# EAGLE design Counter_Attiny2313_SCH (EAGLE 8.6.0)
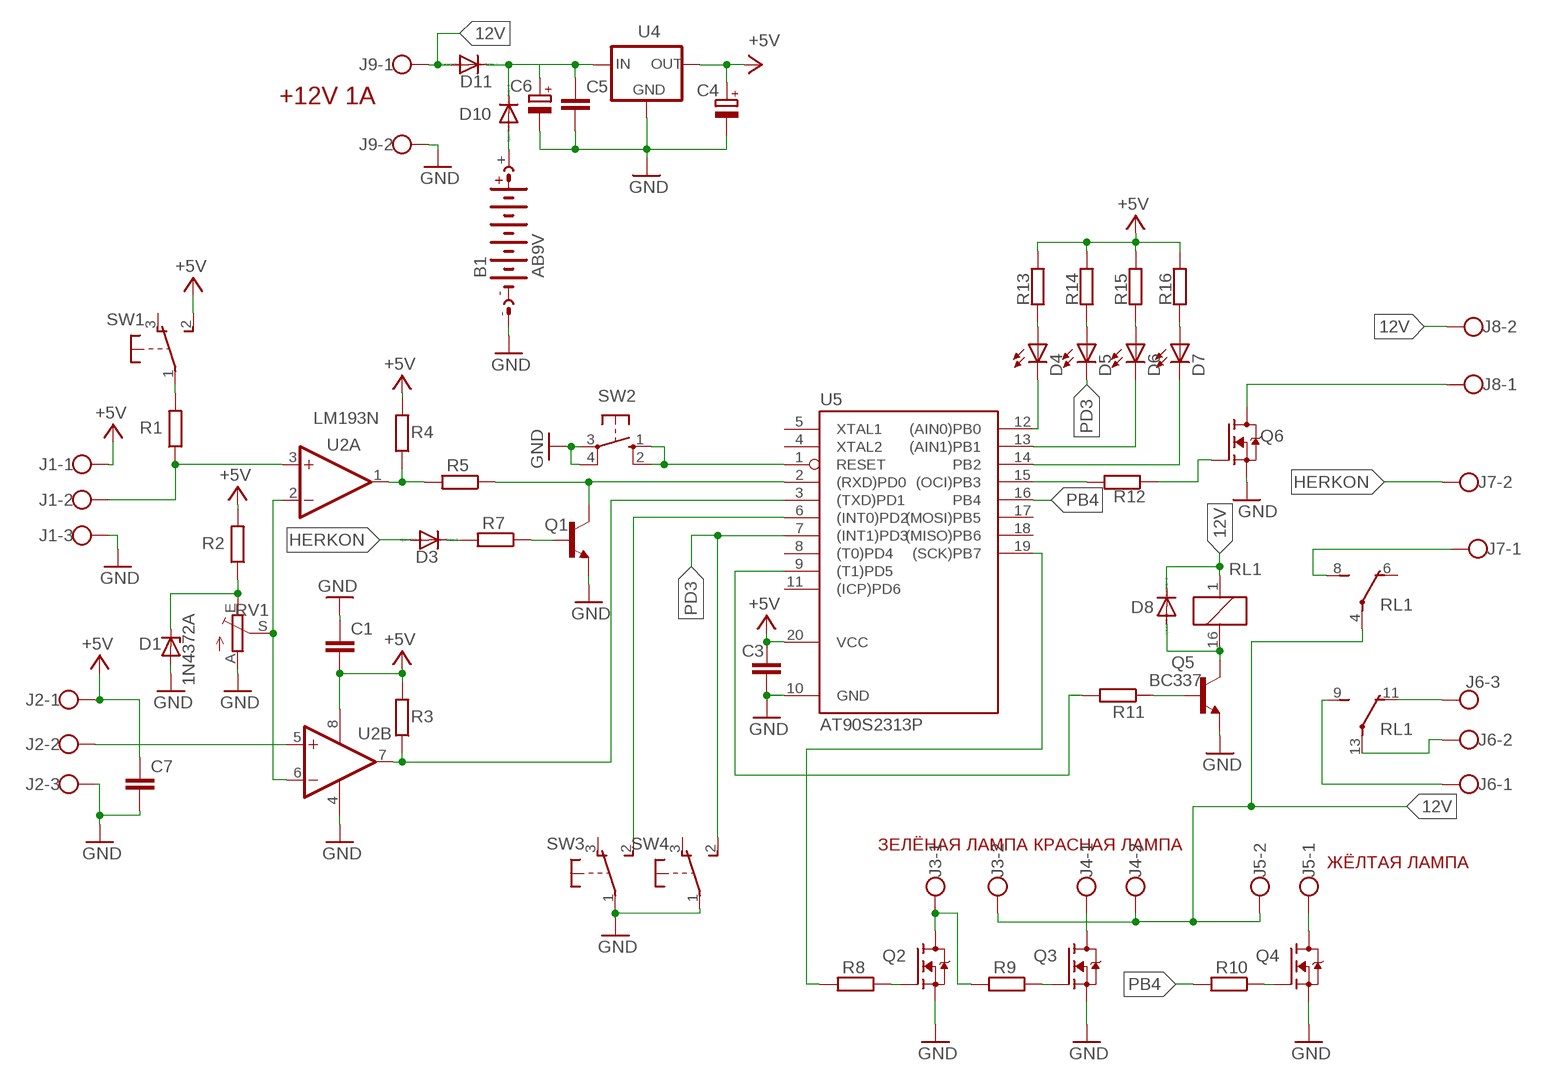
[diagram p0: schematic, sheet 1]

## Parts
B1  AB9V  [AB9V]
C1  C-EUC1206  [C1206]
C3  C-EUC1206  [C1206]
C4  CPOL-EUC/6032-28W  [C/6032-28W]
C5  C-EUC1206  [C1206]
C6  CPOL-EUC/6032-28W  [C/6032-28W]
C7  C-EUC1206  [C1206]
D1  1N4372A  BZX85  [DO41Z10]
D3  1N4148DO35-7  [DO35-7]
D4  LED5MM  [LED5MM]
D5  LED5MM  [LED5MM]
D6  LED5MM  [LED5MM]
D7  LED5MM  [LED5MM]
D8  1N4148DO35-7  [DO35-7]
D10  1N4004  [DO41-10]
D11  1N4004  [DO41-10]
J1  W237-103  [W237-103]
J2  W237-103  [W237-103]
J3  W237-102  [W237-102]
J4  W237-102  [W237-102]
J5  W237-102  [W237-102]
J6  W237-103  [W237-103]
J7  W237-102  [W237-102]
J8  W237-102  [W237-102]
J9  W237-102  [W237-102]
Q1  BC337  [TO92]
Q2  IRL3410  [TO252]
Q3  IRL3410  [TO252]
Q4  IRL3410  [TO252]
Q5  BC337  [TO92]
Q6  IRL3410  [TO252]
R1  R-EU_R1206  [R1206]
R2  R-EU_R1206  [R1206]
R3  R-EU_R1206  [R1206]
R4  R-EU_R1206  [R1206]
R5  R-EU_R1206  [R1206]
R7  R-EU_R1206  [R1206]
R8  R-EU_R1206  [R1206]
R9  R-EU_R1206  [R1206]
R10  R-EU_R1206  [R1206]
R11  R-EU_R1206  [R1206]
R12  R-EU_R1206  [R1206]
R13  R-EU_R1206  [R1206]
R14  R-EU_R1206  [R1206]
R15  R-EU_R1206  [R1206]
R16  R-EU_R1206  [R1206]
RL1  G5V-2  [G5V-2]
RV1  TRIM_EU-CT6  [CT6]
SW1  9077-1  [9077-1]
SW2  10-XX  [B3F-10XX]
SW3  9077-1  [9077-1]
SW4  9077-1  [9077-1]
U2  LM193N  LM393N  [DIL08]
U4  78XXL  [78XXL]
U5  AT90S2313P  [DIL20]

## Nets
12V: D8.C D11.A J3.2 J4.2 J5.2 J8.2 J9.1 RL1.1 RL1.4(1:P)
+5V: C1.2 C3.1 C4.+ C7.1 J1.1 J2.1 R2.2 R3.2 R4.2 R13.2 R14.2 R15.2 R16.2 SW1.2(S) U2.8(P:V+) U4.OUT U5.20(VCC)
GND: B1.- C1.1 C3.2 C4.- C5.2 C6.- C7.2 D1.A J1.3 J2.3 J9.2 Q1.1(E) Q2.3(S) Q3.3(S) Q4.3(S) Q5.1(E) Q6.3(S) RV1.A SW2.3(P) SW2.4(P1) SW3.1(P) SW4.1(P) U2.4(P:V-) U4.GND U5.10(GND)
HERKON: D3.A J7.2
N$1: R1.2 SW1.1(P)
N$2: J1.2 R1.1 U2.3(A:+IN)
N$3: D1.C R2.1 RV1.E
N$4: R3.1 U2.7(B:OUT) U5.3((TXD)PD1)
N$5: RV1.S U2.2(A:-IN) U2.6(B:-IN)
N$6: J2.2 U2.5(B:+IN)
N$7: R4.1 R5.2 U2.1(A:OUT)
N$8: Q1.2(B) R7.1
N$9: D3.C R7.2
N$10: R11.2 U5.9((T1)PD5)
N$11: Q1.3(C) R5.1 U5.2((RXD)PD0)
N$12: SW2.1(S) SW2.2(S1) U5.1(RESET)
N$13: SW3.2(S) U5.6((INT0)PD2)
N$14: J6.1 RL1.9(2:S)
N$15: J4.1 Q3.2(D)
N$16: J3.1 Q2.2(D) R9.2
N$17: Q2.1(G) R8.1
N$19: Q3.1(G) R9.1
N$20: J5.1 Q4.2(D)
N$21: Q4.1(G) R10.1
N$22: R8.2 U5.19((SCK)PB7)
N$24: Q5.2(B) R11.1
N$25: D8.A Q5.3(C) RL1.16
N$26: J6.2 RL1.13(2:P)
N$27: J6.3 RL1.11(2:O)
N$28: R12.2 U5.15((OCI)PB3)
N$29: J7.1 RL1.8(1:S)
N$30: Q6.1(G) R12.1
N$31: J8.1 Q6.2(D)
N$32: D4.A R13.1
N$33: D5.A R14.1
N$34: D6.A R15.1
N$35: D7.A R16.1
N$36: D4.K(C) U5.12((AIN0)PB0)
N$37: D6.K(C) U5.13((AIN1)PB1)
N$38: D7.K(C) U5.14(PB2)
N$39: C5.1 C6.+ D10.C D11.C U4.IN
N$40: B1.+ D10.A
PB4: R10.2 U5.16(PB4)
PD3: D5.K(C) SW4.2(S) U5.7((INT1)PD3)
Unconnected: RL1.6(1:O) SW1.3(O) SW3.3(O) SW4.3(O) U5.4(XTAL2) U5.5(XTAL1) U5.8((T0)PD4) U5.11((ICP)PD6) U5.17((MOSI)PB5) U5.18((MISO)PB6)

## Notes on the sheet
- +12V 1A
- ЗЕЛЁНАЯ ЛАМПА | КРАСНАЯ ЛАМПА
- ЖЁЛТАЯ ЛАМПА

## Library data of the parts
B1 = battery:AB9V: 9-V BATTERY CLIP
C1 C3 C5 C7 = rcl:C-EU: CAPACITOR, European symbol
C4 C6 = rcl:CPOL-EU: POLARIZED CAPACITOR, European symbol
D1 = diode:BZX85: Z DIODE
D3 D8 = diode:1N4148: DIODE
D4-D7 = led:LED: LED
D10 D11 = diode:1N4004: DIODE
J1 J2 J6 = con-wago-500:W237-103: WAGO SCREW CLAMP; MPN: 237-103; OC_FARNELL: unknown; OC_NEWARK: 18M7116
J3-J5 J7-J9 = con-wago-500:W237-102: WAGO SCREW CLAMP; MPN: 237-102; OC_FARNELL: unknown; OC_NEWARK: 70K9898
Q1 Q5 = transistor:BC337: NPN TRANSISTOR
Q2-Q4 Q6 = transistor-fet:IRL3410
R1-R5 R7-R16 = rcl:R-EU_: RESISTOR, European symbol
RL1 = relay:G5V-2: OMRON PCB Relay Source: http://www.omron.com/ecb/products/pdf/en-g5v2.pdf; MPN: G5V-2 5DC; OC_FARNELL: 9949488; OC_NEWARK: 78K5703
RV1 = pot:TRIM_EU-: POTENTIOMETER
SW1 SW3 SW4 = switch-misc:9077-1: MARQUARDT SWITCH 9077.0100 Distributor: Buerklin
SW2 = switch-omron:10-XX: OMRON SWITCH; MPN: B3F-1000; OC_FARNELL: 176432; OC_NEWARK: 36M3542
U2 = linear:LM393: COMPARATOR
U4 = v-reg:78XXL: VOLTAGE REGULATOR
U5 = atmel:AT90S2313: MICROCONTROLLER 2 Kbytes FLASH 128 bytes SRAM 128 bytes EEPROM UART; OC_FARNELL: unknown; OC_NEWARK: unknown

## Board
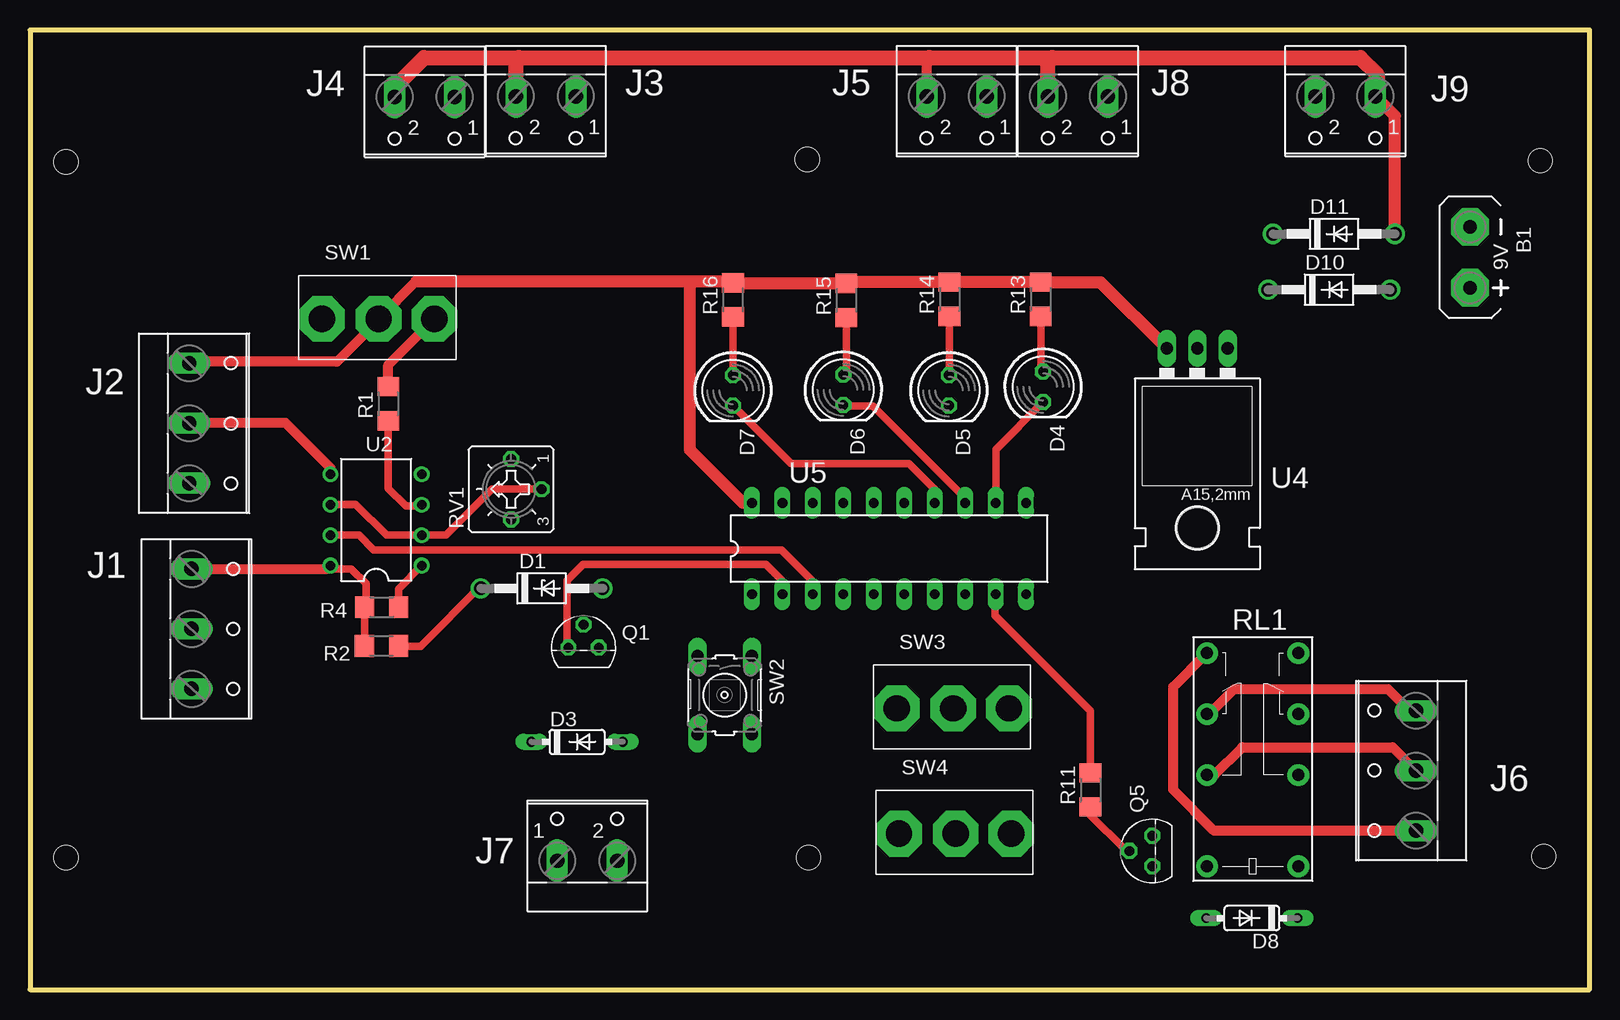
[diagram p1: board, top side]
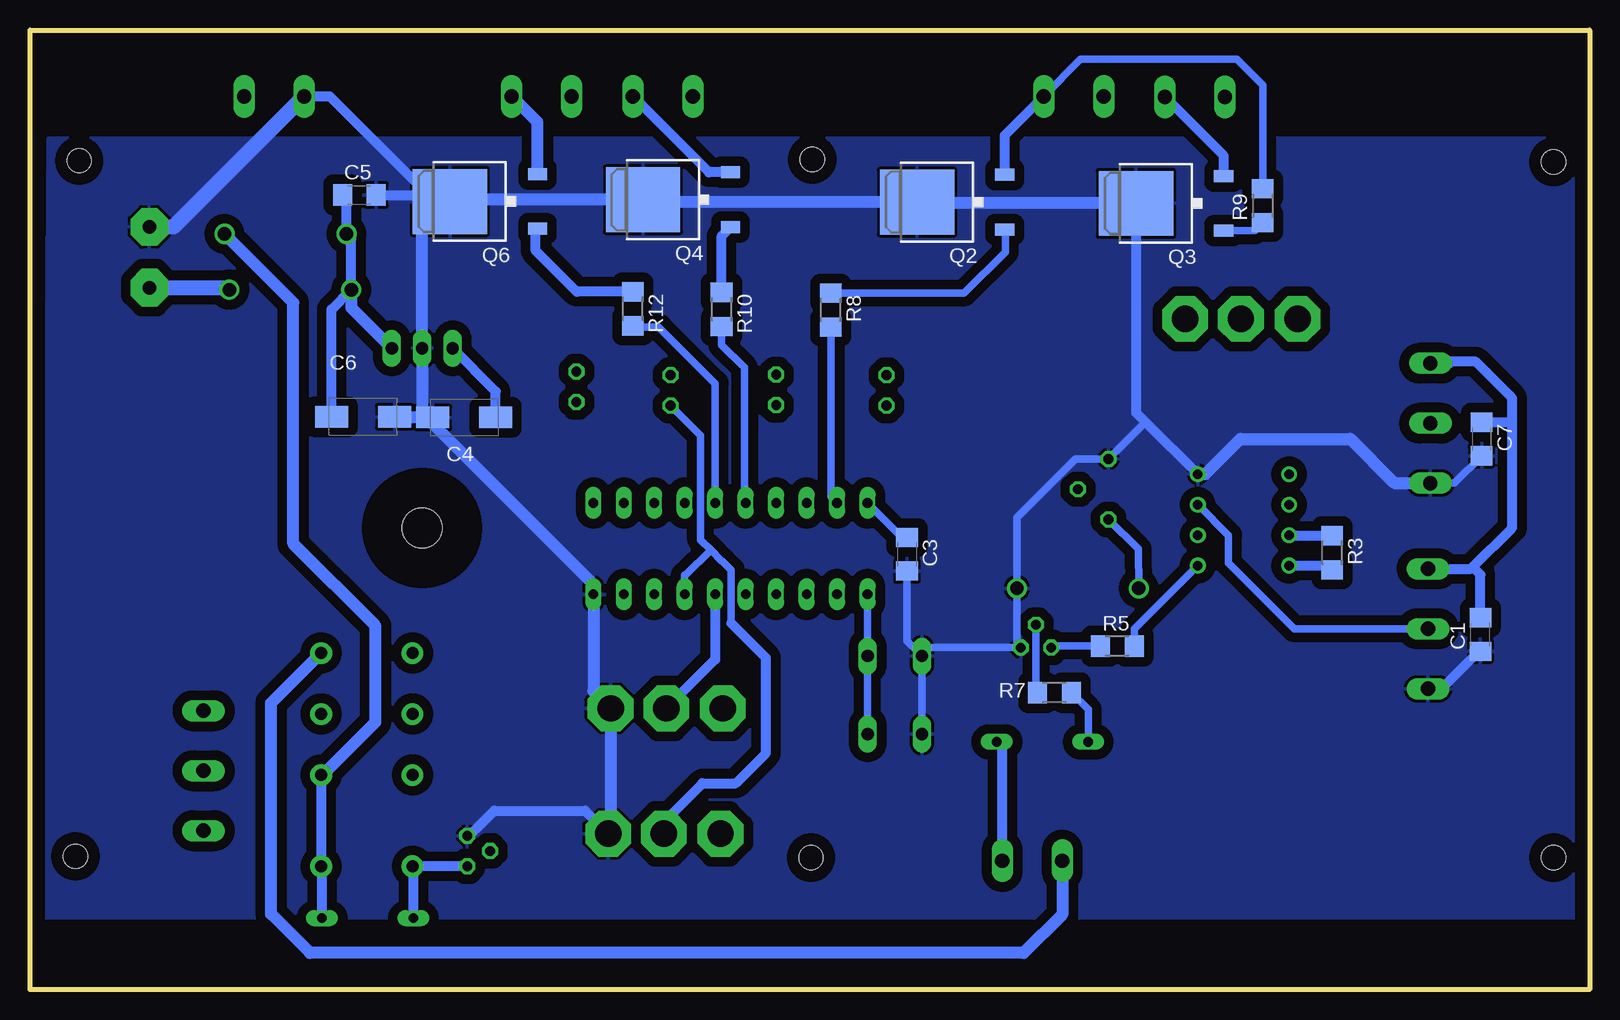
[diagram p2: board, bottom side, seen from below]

Size 130 x 80 mm. Coordinates in mm from the lower left corner, seen from the top.
Outline: 0,0 130,0 130,80 0,80 0,0
Copper layers (1*16): Top 0.035mm / dielectric 1.5mm / Bottom 0.035mm
Design rules "default": minimum track width 10mil, minimum drill 24mil, track to track 8mil, track to pad 8mil, pad to pad 8mil, via to via 8mil, smd to smd 8mil, copper to edge 40mil, drill to drill 8mil, minimum pad ring 10mil, minimum via ring 8mil, stop-mask expansion 4mil, vias tented up to drill 0mil, thermal gap 10mil
Holes 2 mm at 3,69 64.8,69.2 125.9,69.1 3,11 64.9,11 126.2,11.1

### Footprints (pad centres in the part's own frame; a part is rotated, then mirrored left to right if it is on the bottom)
AB9V = drill 1.118 pad 3.15 octagon: + 0,2.54; - 0,-2.54
C1206 = smd 1.6 x 1.8: 1 -1.4,0; 2 1.4,0
C/6032-28W = smd 2.75 x 1.8: + 2.625,0; - -2.625,0
DO41Z10 = drill 1.118: A 5.08,0; C -5.08,0
DO35-7 = drill 0.813 long: A 3.81,0; C -3.81,0
LED5MM = drill 0.813 octagon: A -1.27,0; K 1.27,0
DO41-10 = drill 1.118: A 5.08,0; C -5.08,0
W237-103 = drill 1.194 long: 1 -5,-1.29; 2 0,-1.29; 3 5,-1.29
W237-102 = drill 1.194 long: 1 -2.5,-1.27; 2 2.5,-1.27
TO92 = drill 0.813 octagon: 1 1.27,0; 2 0,1.905; 3 -1.27,0
TO252 = smd 1 x 1.6: 1 -2.28,-4.8; 2 2.28,-4.8 | smd 5.4 x 6.2: 3 0,2.5
R1206 = smd 1.6 x 1.803: 1 -1.422,0; 2 1.422,0
G5V-2 = drill 1 pad 1.8: 1 -8.89,-3.81; 4 -1.27,-3.81; 6 3.81,-3.81; 8 8.89,-3.81; 9 8.89,3.81; 11 3.81,3.81; 13 -1.27,3.81; 16 -8.89,3.81
CT6 = drill 0.813 octagon: A 2.515,0; E -2.515,0; S 0,-2.54
9077-1 = drill 2.2 pad 3.81 octagon: 1 4.7,-0.116; 2 0.06,-0.116; 3 -4.66,-0.116
B3F-10XX = drill 1.016 long: 1 -3.251,2.261; 2 3.251,2.261; 3 -3.251,-2.261; 4 3.251,-2.261
DIL08 = drill 0.813 pad 1.27: 1 -3.81,-3.81; 2 -1.27,-3.81; 3 1.27,-3.81; 4 3.81,-3.81; 5 3.81,3.81; 6 1.27,3.81; 7 -1.27,3.81; 8 -3.81,3.81
78XXL = drill 1.016 long: GND 0,-3.81; IN -2.54,-3.81; OUT 2.54,-3.81 | hole 3.302: 0,11.176
DIL20 = drill 0.813 long: 1 -11.43,-3.81; 2 -8.89,-3.81; 3 -6.35,-3.81; 4 -3.81,-3.81; 5 -1.27,-3.81; 6 1.27,-3.81; 7 3.81,-3.81; 8 6.35,-3.81; 9 8.89,-3.81; 10 11.43,-3.81; 11 11.43,3.81; 12 8.89,3.81; 13 6.35,3.81; 14 3.81,3.81; 15 1.27,3.81; 16 -1.27,3.81; 17 -3.81,3.81; 18 -6.35,3.81; 19 -8.89,3.81; 20 -11.43,3.81

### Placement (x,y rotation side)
B1  120.05,61.05 180 top
C1  9.1,29.6 90 bottom
C3  56.9,36.29 270 bottom
C4  93.8,47.7 0 bottom
C5  102.55,66.25 0 bottom
C6  102.25,47.75 180 bottom
C7  9,45.9 270 bottom
D1  42.65,33.45 0 top
D3  45.6,20.65 0 top
D4  84.45,50.25 270 top
D5  76.6,49.95 270 top
D6  67.8,50 270 top
D7  58.6,49.95 270 top
D8  101.85,5.95 180 top
D10  108.3,58.35 0 top
D11  108.7,63 0 top
J1  14.76,30.07 270 top
J2  14.56,47.21 270 top
J3  43,73.2 180 top
J4  32.9,73.15 180 top
J5  77.25,73.2 180 top
J6  114.25,18.25 90 top
J7  46.45,12 0 top
J8  87.35,73.2 180 top
J9  109.65,73.2 180 top
Q1  46.14,28.51 0 top
Q2  53.55,65.65 90 bottom
Q3  35.3,65.55 90 bottom
Q4  76.4,65.85 90 bottom
Q5  93.55,11.55 90 top
Q6  92.5,65.7 90 bottom
R1  29.86,48.84 90 top
R2  29.3,28.65 180 top
R3  21.45,36.41 270 bottom
R4  29.31,31.88 180 top
R5  39.36,28.64 0 bottom
R7  44.61,24.75 0 bottom
R8  63.25,56.65 270 bottom
R9  27.25,65.35 90 bottom
R10  72.35,56.7 270 bottom
R11  88.4,16.65 90 top
R12  79.75,56.75 270 bottom
R13  84.25,57.55 90 top
R14  76.65,57.55 90 top
R15  68.05,57.45 90 top
R16  58.6,57.5 90 top
RL1  101.92,19.16 90 top
RV1  40.1,41.71 90 top
SW1  29,56.03 0 top
SW2  57.91,24.55 270 top
SW3  76.9,23.55 0 top
SW4  77.1,13.1 0 top
U2  28.85,39.15 90 top
U4  97.3,49.65 180 top
U5  71.61,36.76 0 top

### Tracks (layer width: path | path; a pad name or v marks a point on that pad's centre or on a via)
12V
  Top 0.813: J5.2 74.75,77.5 74.95,77.7
  Top 1.016: D11.A 113.78,72.84 J9.1
  Top 1.27: J4.2 30.4,75.25 32.85,77.7 40.75,77.7 | 40.75,77.7 74.95,77.7 85.2,77.7 | 85.2,77.7 110.9,77.7 112.3,76.3 112.3,74.62 J9.1 | J8.2 84.85,77.35 85.2,77.7 | J3.2 40.5,77.45 40.75,77.7
  Bottom 0.813: D8.C 105.66,10.2 RL1.1 RL1.4
  Bottom 1.016: RL1.4 105.61,17.89 101.2,22.3 101.2,30.3 108.05,37.15 108.05,57.27 D11.A
+5V
  Top 0.61: R2.2 27.88,31.87 R4.2 28,31.99 28,33.85 26.78,35.07 24.77,35.07
  Top 0.813: 29.06,55.81 SW1.2 32.2,59.05 | 29.06,55.81 25.6,52.35 13.41,52.35 J2.1 | 29.1,55.85 29.06,55.81 | J1.1 24.77,35.07 U2.8
  Top 1.016: 32.2,59.05 55,59.05 | 55,59.05 58.47,59.05 R16.2 58.65,58.87 R15.2 68.15,58.97 R14.2 R13.2 89.25,58.97 U4.OUT | U5.20 59.43,40.57 55,45 55,59.05
  Bottom 0.61: C3.1 57.3,37.69 U5.20
  Bottom 0.813: 11.65,52.2 12.7,52.2 | 12.7,52.2 J2.1 | U2.8 21.8,35.34 R3.2 | 6.45,47.5 6.45,38.5 9.72,35.23 | 6.45,47.5 6.45,49.3 9.5,52.35 12.55,52.35 12.7,52.2 | C7.1 6.65,47.3 6.45,47.5 | J1.1 9.88,35.07 9.72,35.23 | C1.2 9.1,34.6 9.72,35.23 | C4.+ 91.17,49.88 U4.OUT
GND
  Bottom 0.61: J2.3 11.29,42.21 C7.2 | SW2.3 54.94,28.51 Q1.1 47.73,28.83 D1.A 47.73,39.37 42.85,44.25 40.12,44.25 RV1.A 40.1,44.25 37.02,47.33 | SW2.3 SW2.4 | C3.2 56.9,29.05 SW2.3
  Bottom 0.813: Q3.3 37.8,48.1 37.02,47.33 U2.4 | C1.1 9.22,28.2 12.35,25.07 J1.3 | Q5.1 93.38,12.82 91.3,14.9 83.72,14.9 SW4.1 | C5.2 97.35,66.25 96.9,65.8 96.35,65.8 | 96.35,65.8 95.65,65.8 95.42,66.03 | J9.2 105.02,74.47 96.35,65.8
  Bottom 1.016: U2.4 32.04,42.96 29.1,45.9 19.95,45.9 16.3,42.25 13.31,42.25 J2.3 | SW4.1 81.6,13.18 SW3.1 83.04,24.87 U5.10 83.04,33.79 96.95,47.7 | Q3.3 55.95,65.55 Q2.3 79.15,65.65 79.4,65.9 78.95,65.9 Q4.3 95.25,65.85 | 95.25,65.85 95.42,66.03 95.55,66.15 | 95.25,65.85 95.1,65.7 Q6.3 97.3,63.4 U4.GND 97.3,48.05 96.95,47.7 | C4.- 96.95,47.7 | 96.95,47.7 99.58,47.7 C6.-
  Bottom 1.27: B1.- 118.03,63.59 J9.2
  pour Bottom (isolate 0.813): 1,71 128.5,71 129,6 1,6
HERKON
  Bottom 0.813: J7.2 48.95,20.19 D3.A
N$1
  Top 0.813: R1.2 29.86,52.07 SW1.1
N$2
  Top 0.61: R1.1 29.86,41.79 31.35,40.3 32.54,40.3 U2.3
  Bottom 0.61: J1.2 24.62,30.07 30.1,35.55 30.1,37.86 U2.3
N$3
  Top 0.61: D1.C 37.62,33.67 32.55,28.6 30.77,28.6 R2.1
  Bottom 0.61: D1.C 37.62,36.72 RV1.E
N$4
  Top 0.61: U2.7 27.42,37.88 28.65,36.65 62.65,36.65 65.2,34.1 65.2,33.01 U5.3
  Bottom 0.813: R3.1 24.99,37.83 U2.7
N$5
  Top 0.61: U2.6 25.07,40.45 27.15,40.45 29.72,37.88 U2.2 32.68,37.9 34.7,37.9 38.51,41.71 RV1.S
N$6
  Top 0.813: U2.5 25.04,43.51 21.3,47.25 13.31,47.25 J2.2
N$7
  Top 0.61: R4.1 30.73,33.41 U2.1
  Bottom 0.61: R5.2 37.94,30.06 U2.1
N$8
  Bottom 0.61: Q1.2 46.14,24.86 R7.1
N$9
  Bottom 0.61: D3.C 41.79,23.35 R7.2
N$10
  Top 0.61: R11.2 88.4,23.25 80.45,31.2 80.45,32.9 U5.9
N$11
  Top 0.61: U5.2 62.72,34.08 61.35,35.45 46.1,35.45 44.75,34.1 44.75,28.63 Q1.3
  Bottom 0.61: R5.1 44.74,28.64 Q1.3
N$12
  Bottom 0.61: U5.1 SW2.1 SW2.2
N$13
  Bottom 0.813: U5.6 72.88,27.51 SW3.2
N$14
  Top 0.813: J6.1 98.7,13.25 95.3,16.65 95.3,25.24 RL1.9
N$15
  Bottom 0.813: Q3.2 30.5,69.52 J4.1
N$16
  Bottom 0.61: R9.2 27.25,75.4 29.4,77.55 42.42,77.55 J3.1
  Bottom 0.813: Q2.2 48.75,71.22 J3.1
N$17
  Bottom 0.61: R8.1 52.13,58.07 48.7,61.5 48.7,63.32 Q2.1
N$19
  Bottom 0.61: Q3.1 27.91,63.27 R9.1
N$20
  Bottom 0.813: Q4.2 73.41,68.13 J5.1
N$21
  Bottom 0.813: R10.1 72.35,62.82 Q4.1
N$22
  Bottom 0.61: R8.2 63.25,41.1 U5.19
N$24
  Top 0.61: Q5.2 91.4,11.55 88.2,14.75 88.2,15.03 R11.1
N$25
  Bottom 0.813: Q5.3 RL1.16 98.04,10.2 D8.A
N$26
  Top 0.813: RL1.13 98.74,17.89 101.05,20.2 113.59,20.2 J6.2
N$27
  Top 0.813: RL1.11 98.32,22.97 100.4,25.05 113.2,25.05 115,23.25 J6.3
N$28
  Bottom 0.61: U5.15 72.88,50.53 77.6,55.25 79.67,55.25 R12.2
N$29
  Bottom 1.016: J7.1 43.95,6.25 47.15,3.05 106.65,3.05 109.9,6.3 109.9,23.88 RL1.8
N$30
  Bottom 0.813: R12.1 84.42,58.17 87.85,61.6 87.85,63.27 Q6.1
N$31
  Bottom 1.016: Q6.2 87.7,72.32 J8.1
N$32
  Top 0.61: R13.1 84.25,51.72 D4.A
N$33
  Top 0.61: R14.1 76.65,51.27 D5.A
N$34
  Top 0.61: R15.1 68.05,51.52 D6.A
N$35
  Top 0.61: D7.A R16.1
N$36
  Top 0.61: U5.12 80.5,45.03 D4.K
N$37
  Top 0.61: U5.13 77.96,40.94 70.25,48.65 67.88,48.65 D6.K
N$38
  Top 0.61: U5.14 75.42,41.68 73.25,43.85 63.43,43.85 D7.K
N$39
  Bottom 0.813: C6.+ 104.88,56.7 D10.C 103.22,62.6 D11.C 103.62,65.92 C5.1
  Bottom 1.016: D10.C 103.22,56.84 U4.IN
N$40
  Bottom 1.27: B1.+ 113.54,58.51 D10.A
PB4
  Bottom 0.61: R10.2 72.35,53.75 70.45,51.85 70.45,40.68 U5.16
PD3
  Bottom 0.61: U5.7 75.45,32.98 75.45,34.55 75.35,34.55 73.25,36.65 | 71.55,30.55 71.55,35 72.3,35.75 72.35,35.75 73.25,36.65 | 73.25,36.65 74.1,37.5 74.1,46.18 D5.K
  Bottom 0.813: SW4.2 77.16,13.99 73.95,17.2 71.15,17.2 68.65,19.7 68.65,27.65 71.55,30.55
